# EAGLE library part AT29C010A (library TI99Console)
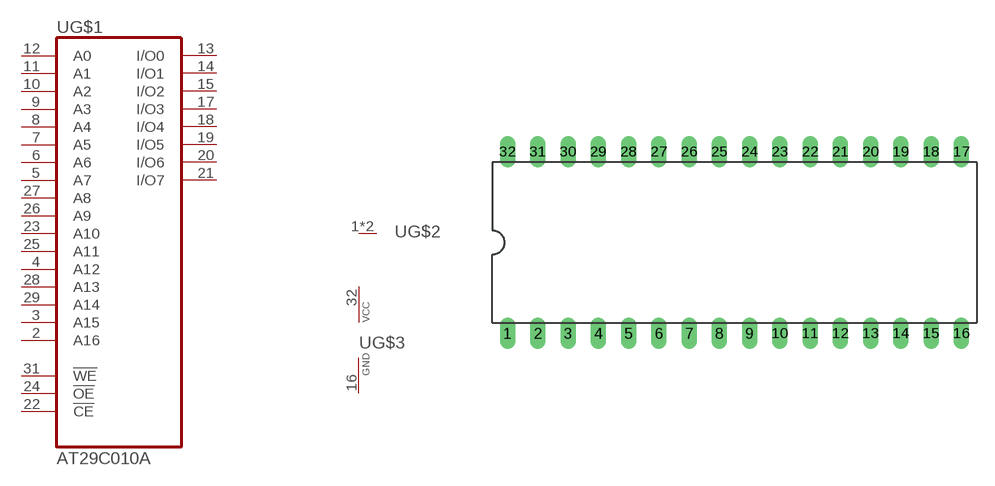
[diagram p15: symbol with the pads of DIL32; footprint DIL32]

Designator prefix -; gates G$1=AT29C010A G$2=NC G$3=VCC-GND

## AT29C010A-DIL32  [DIL32]
1  G$2:NC  nc
2  G$1:A16  in
3  G$1:A15  in
4  G$1:A12  in
5  G$1:A7  in
6  G$1:A6  in
7  G$1:A5  in
8  G$1:A4  in
9  G$1:A3  in
10  G$1:A2  in
11  G$1:A1  in
12  G$1:A0  in
13  G$1:I/O0
14  G$1:I/O1
15  G$1:I/O2
16  G$3:GND  pwr
17  G$1:I/O3
18  G$1:I/O4
19  G$1:I/O5
20  G$1:I/O6
21  G$1:I/O7
22  G$1:!CE  in
23  G$1:A10  in
24  G$1:!OE  in
25  G$1:A11  in
26  G$1:A9  in
27  G$1:A8  in
28  G$1:A13  in
29  G$1:A14  in
30  G$2:NC  nc
31  G$1:!WE  in
32  G$3:VCC  pwr

## Footprint DIL32 (pad centres in mm)
Dual In Line Package
drill 0.813 long: 1 -19.05,-7.62; 2 -16.51,-7.62; 3 -13.97,-7.62; 4 -11.43,-7.62; 5 -8.89,-7.62; 6 -6.35,-7.62; 7 -3.81,-7.62; 8 -1.27,-7.62; 9 1.27,-7.62; 10 3.81,-7.62; 11 6.35,-7.62; 12 8.89,-7.62; 13 11.43,-7.62; 14 13.97,-7.62; 15 16.51,-7.62; 16 19.05,-7.62; 17 19.05,7.62; 18 16.51,7.62; 19 13.97,7.62; 20 11.43,7.62; 21 8.89,7.62; 22 6.35,7.62; 23 3.81,7.62; 24 1.27,7.62; 25 -1.27,7.62; 26 -3.81,7.62; 27 -6.35,7.62; 28 -8.89,7.62; 29 -11.43,7.62; 30 -13.97,7.62; 31 -16.51,7.62; 32 -19.05,7.62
